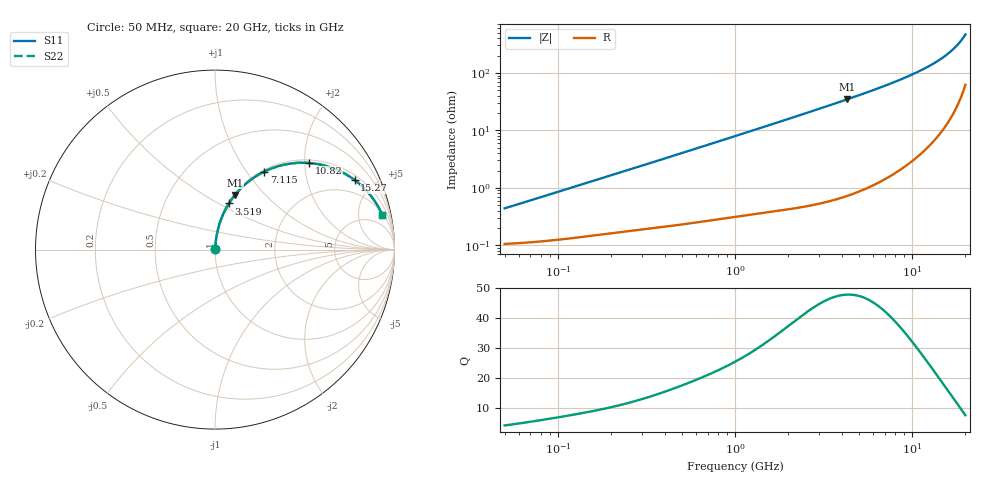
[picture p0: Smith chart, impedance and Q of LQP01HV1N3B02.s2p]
!Murata Part Number: LQP01HV1N3B02
!These Parameters are Measured in Series Mode Connection
!  o--[Z]--o
!Port1  Port2
!  o-------o
!Freq. Start=50[MHz] Stop=20[GHz], 401[Steps]
# Hz S RI R 50
!Freq.(Hz) S11(Real) S11(Imag) S21(Real) S21(Imag) S12(Real) S12(Imag) S22(Real) S22(Imag)
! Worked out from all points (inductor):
!   401 points, 50 MHz to 20 GHz, reference 50 ohm
!   read as one part in series: L = 1.35 nH near 51.52 MHz
!   highest Q = 47.9 at 4.276 GHz (marker M1), where L = 1.28 nH
!   S11 on the Smith chart (normalised r, x): 50 MHz: 1.00, +0.01; 3.519 GHz: 1.01, +0.56; 7.115 GHz: 1.03, +1.21; 10.82 GHz: 1.07, +2.10; 15.27 GHz: 1.23, +3.89; 20 GHz: 2.24, +9.24
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5e7  0.00107 0.00425  0.9989 -0.00425  0.9989 -0.00425  0.00107 0.00425
1.364002e8  0.00152 0.0113  0.9985 -0.0113  0.9985 -0.0113  0.00152 0.0113
3.721004e8  0.00294 0.0299  0.9971 -0.0299  0.9971 -0.0299  0.00294 0.0299
6.380365e8  0.00512 0.0505  0.9949 -0.0505  0.9949 -0.0505  0.00512 0.0505
1e9  0.00929 0.0782  0.9907 -0.0782  0.9907 -0.0782  0.00929 0.0782
1.714689e9  0.0217 0.1318  0.9783 -0.1318  0.9783 -0.1318  0.0217 0.1318
2.728004e9  0.0489 0.2044  0.9511 -0.2044  0.9511 -0.2044  0.0489 0.2044
3.519108e9  0.0777 0.2573  0.9223 -0.2573  0.9223 -0.2573  0.0777 0.2573
4.275624e9  0.111 0.3038  0.889 -0.3038  0.889 -0.3038  0.111 0.3038
5.598765e9  0.1805 0.374  0.8195 -0.374  0.8195 -0.374  0.1805 0.374
7.114996e9  0.2735 0.434  0.7265 -0.434  0.7265 -0.434  0.2735 0.434
7.442007e9  0.2949 0.4439  0.7051 -0.4439  0.7051 -0.4439  0.2949 0.4439
9.178299e9  0.412 0.4781  0.588 -0.4781  0.588 -0.4781  0.412 0.4781
1.082228e10  0.523 0.4828  0.477 -0.4828  0.477 -0.4828  0.523 0.4828
1.295331e10  0.6565 0.4538  0.3435 -0.4538  0.3435 -0.4538  0.6565 0.4538
1.417136e10  0.7241 0.4227  0.2759 -0.4227  0.2759 -0.4227  0.7241 0.4227
1.527346e10  0.7784 0.3874  0.2216 -0.3874  0.2216 -0.3874  0.7784 0.3874
1.646126e10  0.8293 0.3435  0.1707 -0.3435  0.1707 -0.3435  0.8293 0.3435
1.747767e10  0.8662 0.3024  0.1338 -0.3024  0.1338 -0.3024  0.8662 0.3024
1.828096e10  0.8912 0.2684  0.1088 -0.2684  0.1088 -0.2684  0.8912 0.2684
1.940974e10  0.92 0.219  0.08 -0.219  0.08 -0.219  0.92 0.219
2e10  0.9324 0.1928  0.0676 -0.1928  0.0676 -0.1928  0.9324 0.1928
